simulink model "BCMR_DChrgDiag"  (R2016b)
settings: Solver=FixedStepDiscrete  StartTime=0.0  StopTime=10  FixedStep=0.01  RelTol=1e-3  EnableMultiTasking=on
undefined symbols (not defined in the file or in its folder): BCMR_bDChrgStopCActiveSw_C, BCMR_cntDChrgTCnntMax_C, BCMR_cntIsoFltTrigger_CW, BCMR_EVCCDiagccSw_C, BCMR_EVCCDiagSw_C, BCMR_G1E0PlatformSwDiag_C, BCMR_H1U0PlatformSwDiag_C, BCMR_iDcChrgDiffOvrCurr_C, BCMR_iDcChrgLowTempDiffOvrCurrMody_C, BCMR_iDcChrgLowTempOvrCurrCutOff_C, BCMR_iDcChrgLowTempOvrCurrHeal_C, BCMR_iDcChrgOvrCurr_C, BCMR_iDcChrgOvrVolt_C, BCMR_iDChrgCurrDiagLmt_C, BCMR_iDChrgCutOffVoltOvrCurrDet_C, BCMR_iDChrgCutOffVoltOvrCurrHeal_C, BCMR_kWaveFltFactor_C, BCMR_stCCSTimeout_C, BCMR_stCHMTimeout_C, BCMR_stCMLTimeout_C, BCMR_stCRMAATimeout_C, BCMR_stCROAATimeout_C, BCMR_stCROTimeout_C, BCMR_stCSDTimeout1_C, BCMR_stCSDTimeout2_C, BCMR_stCSTTimeout_C, BCMR_stCurrDwnTimeout_C, BCMR_stHvOnTimeout_C, BCMR_stNoTimeout_C, BCMR_stParaMish_C, BCMR_tBattLowTempDiagTempThrd_C, BCMR_tDcChrgIntfTempDiffLmt_C, BCMR_tDcChrgIntfTempLmt_C, BCMR_tiDChrgDetDiagDebs_C, BCMR_tiDChrgDetSec_C, BCMR_tiDChrgDiagBase_C, BCMR_tiDChrgHealDiagDebs_C, BCMR_tiDChrgIntfTempDwnLmt_C, BCMR_tiDChrgLowTOvrCurrDet_C, BCMR_tiDChrgLowTOvrCurrHeal_C, BCMR_tiDChrgMishCurrDetDiagDebs_C, BCMR_tiDChrgOvrCellVolt_C, BCMR_tiDChrgOvrSafeCellVoltDet_C, BCMR_tiDChrgVoltFltDetDebs_C, BCMR_tiDChrgVoltFltHealDebs_C, BCMR_uCC2ChkDiffDet_C, BCMR_uCC2ChkDiffHeal_C, BCMR_uCC2VoltHighDet_C, BCMR_uCC2VoltHighHeal_C, BCMR_uCC2VoltLowDet_C, BCMR_uCC2VoltLowHeal_C, BCMR_uDChrgHighTempDet_C, BCMR_uDChrgHighTempHeal_C, BCMR_uDChrgLowTempDet_C, BCMR_uDChrgLowTempHeal_C, BCMR_uDChrgOvrCellVoltDet_C, BCMR_uDChrgOvrCellVoltHeal_C, BCMR_uDChrgOvrSafeCellVoltDet_C, BCMR_uDChrgOvrSafeCellVoltHeal_C, bin2dec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
libraries: simulink x291
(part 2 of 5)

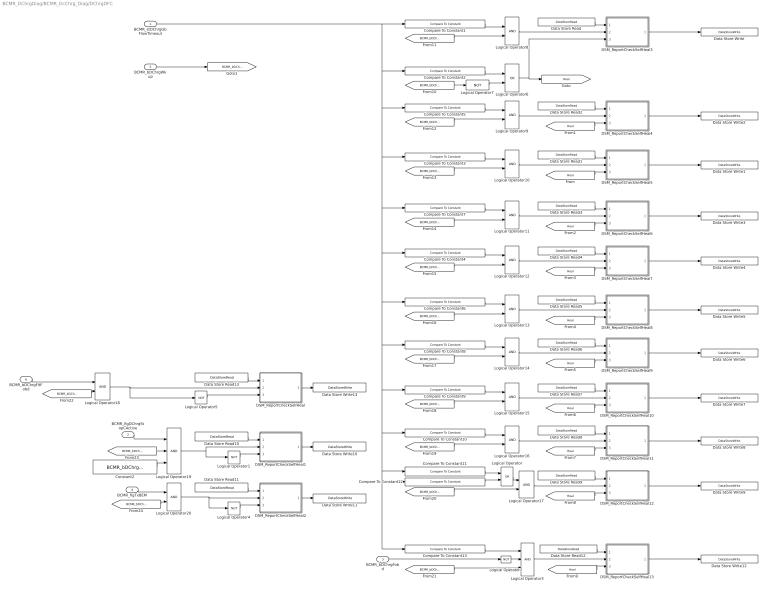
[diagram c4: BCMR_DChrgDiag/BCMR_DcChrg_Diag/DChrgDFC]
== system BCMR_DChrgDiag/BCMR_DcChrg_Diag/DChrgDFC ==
  BCMR_stDChrgGbFlowTimeout : Inport
  BCMR_flgDChrgStopCActive : Inport  Port=2
  BCMR_bDChrgFobd : Inport  Port=3
  BCMR_flgTxBEM : Inport  Port=4
  BCMR_bDChrgWkup : Inport  Port=5
  BCMR_bDChrgFltFobd : Inport  Port=6
  Compare To Constant1 : simulink/Logic and Bit Operations/Compare To Constant  relop===  const=BCMR_stCHMTimeout_C  OutDataTypeStr=boolean
  Compare To Constant10 : simulink/Logic and Bit Operations/Compare To Constant  relop===  const=BCMR_stCurrDwnTimeout_C  OutDataTypeStr=boolean
  Compare To Constant11 : simulink/Logic and Bit Operations/Compare To Constant  relop===  const=BCMR_stCSDTimeout1_C  OutDataTypeStr=boolean
  Compare To Constant12 : simulink/Logic and Bit Operations/Compare To Constant  relop===  const=BCMR_stCSDTimeout2_C  OutDataTypeStr=boolean
  Compare To Constant13 : simulink/Logic and Bit Operations/Compare To Constant  relop===  const=BCMR_stParaMish_C  OutDataTypeStr=boolean
  Compare To Constant2 : simulink/Logic and Bit Operations/Compare To Constant  relop===  const=BCMR_stNoTimeout_C  OutDataTypeStr=boolean
  Compare To Constant3 : simulink/Logic and Bit Operations/Compare To Constant  relop===  const=BCMR_stCRMAATimeout_C  OutDataTypeStr=boolean
  Compare To Constant4 : simulink/Logic and Bit Operations/Compare To Constant  relop===  const=BCMR_stCROTimeout_C  OutDataTypeStr=boolean
  Compare To Constant5 : simulink/Logic and Bit Operations/Compare To Constant  relop===  const=BCMR_stCMLTimeout_C  OutDataTypeStr=boolean
  Compare To Constant6 : simulink/Logic and Bit Operations/Compare To Constant  relop===  const=BCMR_stCROAATimeout_C  OutDataTypeStr=boolean
  Compare To Constant7 : simulink/Logic and Bit Operations/Compare To Constant  relop===  const=BCMR_stHvOnTimeout_C  OutDataTypeStr=boolean
  Compare To Constant8 : simulink/Logic and Bit Operations/Compare To Constant  relop===  const=BCMR_stCCSTimeout_C  OutDataTypeStr=boolean
  Compare To Constant9 : simulink/Logic and Bit Operations/Compare To Constant  relop===  const=BCMR_stCSTTimeout_C  OutDataTypeStr=boolean
  Constant2 : Constant  Value=BCMR_bDChrgStopCActiveSw_C
  DSM_ReportCheckSelfHeal : Subsystem  TreatAsAtomicUnit=on  RTWFcnName=DSM_ReportCheck  RTWFileName=SrvLib
  DSM_ReportCheckSelfHeal1 : Subsystem  TreatAsAtomicUnit=on  RTWFcnName=DSM_ReportCheck  RTWFileName=SrvLib
  DSM_ReportCheckSelfHeal10 : Subsystem  TreatAsAtomicUnit=on  RTWFcnName=DSM_ReportCheck  RTWFileName=SrvLib
  DSM_ReportCheckSelfHeal11 : Subsystem  TreatAsAtomicUnit=on  RTWFcnName=DSM_ReportCheck  RTWFileName=SrvLib
  DSM_ReportCheckSelfHeal12 : Subsystem  TreatAsAtomicUnit=on  RTWFcnName=DSM_ReportCheck  RTWFileName=SrvLib
  DSM_ReportCheckSelfHeal13 : Subsystem  TreatAsAtomicUnit=on  RTWFcnName=DSM_ReportCheck  RTWFileName=SrvLib
  DSM_ReportCheckSelfHeal2 : Subsystem  TreatAsAtomicUnit=on  RTWFcnName=DSM_ReportCheck  RTWFileName=SrvLib
  DSM_ReportCheckSelfHeal3 : Subsystem  TreatAsAtomicUnit=on  RTWFcnName=DSM_ReportCheck  RTWFileName=SrvLib
  DSM_ReportCheckSelfHeal4 : Subsystem  TreatAsAtomicUnit=on  RTWFcnName=DSM_ReportCheck  RTWFileName=SrvLib
  DSM_ReportCheckSelfHeal5 : Subsystem  TreatAsAtomicUnit=on  RTWFcnName=DSM_ReportCheck  RTWFileName=SrvLib
  DSM_ReportCheckSelfHeal6 : Subsystem  TreatAsAtomicUnit=on  RTWFcnName=DSM_ReportCheck  RTWFileName=SrvLib
  DSM_ReportCheckSelfHeal7 : Subsystem  TreatAsAtomicUnit=on  RTWFcnName=DSM_ReportCheck  RTWFileName=SrvLib
  DSM_ReportCheckSelfHeal8 : Subsystem  TreatAsAtomicUnit=on  RTWFcnName=DSM_ReportCheck  RTWFileName=SrvLib
  DSM_ReportCheckSelfHeal9 : Subsystem  TreatAsAtomicUnit=on  RTWFcnName=DSM_ReportCheck  RTWFileName=SrvLib
  Data Store Read : DataStoreRead  DataStoreName=DFC_DChrgCHMTmt
  Data Store Read1 : DataStoreRead  DataStoreName=DFC_DChrgCRMTmt
  Data Store Read10 : DataStoreRead  DataStoreName=DFC_DChrgStakeErr
  Data Store Read11 : DataStoreRead  DataStoreName=DFC_DChrgMsgTmt
  Data Store Read12 : DataStoreRead  DataStoreName=DFC_DChrgParaChk
  Data Store Read13 : DataStoreRead  DataStoreName=DFC_DChrgFobd
  Data Store Read2 : DataStoreRead  DataStoreName=DFC_DChrgCMLTmt
  Data Store Read3 : DataStoreRead  DataStoreName=DFC_DChrgHvOnFail
  Data Store Read4 : DataStoreRead  DataStoreName=DFC_DChrgCROTmt
  Data Store Read5 : DataStoreRead  DataStoreName=DFC_DChrgStkVoltErr
  Data Store Read6 : DataStoreRead  DataStoreName=DFC_DChrgCCSTmt
  Data Store Read7 : DataStoreRead  DataStoreName=DFC_DChrgCSTTmt
  Data Store Read8 : DataStoreRead  DataStoreName=DFC_DChrgStkCurrErr
  Data Store Read9 : DataStoreRead  DataStoreName=DFC_DChrgCSDTmt
  Data Store Write : DataStoreWrite  DataStoreName=DFC_DChrgCHMTmt
  Data Store Write1 : DataStoreWrite  DataStoreName=DFC_DChrgCRMTmt
  Data Store Write10 : DataStoreWrite  DataStoreName=DFC_DChrgStakeErr
  Data Store Write11 : DataStoreWrite  DataStoreName=DFC_DChrgMsgTmt
  Data Store Write12 : DataStoreWrite  DataStoreName=DFC_DChrgParaChk
  Data Store Write13 : DataStoreWrite  DataStoreName=DFC_DChrgFobd
  Data Store Write2 : DataStoreWrite  DataStoreName=DFC_DChrgCMLTmt
  Data Store Write3 : DataStoreWrite  DataStoreName=DFC_DChrgHvOnFail
  Data Store Write4 : DataStoreWrite  DataStoreName=DFC_DChrgCROTmt
  Data Store Write5 : DataStoreWrite  DataStoreName=DFC_DChrgStkVoltErr
  Data Store Write6 : DataStoreWrite  DataStoreName=DFC_DChrgCCSTmt
  Data Store Write7 : DataStoreWrite  DataStoreName=DFC_DChrgCSTTmt
  Data Store Write8 : DataStoreWrite  DataStoreName=DFC_DChrgStkCurrErr
  Data Store Write9 : DataStoreWrite  DataStoreName=DFC_DChrgCSDTmt
  Logical Operator : Logic  Operator=OR  AllPortsSameDT=off  OutDataTypeStr=boolean
  Logical Operator{1..2,4..5,7} (5 alike) : Logic  Operator=NOT  AllPortsSameDT=off  OutDataTypeStr=boolean
  Logical Operator{8..18,20} (12 alike) : Logic  AllPortsSameDT=off  OutDataTypeStr=boolean
  Logical Operator19 : Logic  Inputs=3  AllPortsSameDT=off  OutDataTypeStr=boolean
  Logical Operator3 : Logic  Inputs=3  AllPortsSameDT=off  OutDataTypeStr=boolean
  Logical Operator6 : Logic  Operator=OR  AllPortsSameDT=off  OutDataTypeStr=boolean
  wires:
  DSM_ReportCheckSelfHeal3/1(Dfc_id) -> Data Store Write/1
  Data Store Read/1 -> DSM_ReportCheckSelfHeal3/1(Dfc_id_nv)
  DSM_ReportCheckSelfHeal5/1(Dfc_id) -> Data Store Write1/1
  Data Store Read1/1 -> DSM_ReportCheckSelfHeal5/1(Dfc_id_nv)
  DSM_ReportCheckSelfHeal4/1(Dfc_id) -> Data Store Write2/1
  DSM_ReportCheckSelfHeal6/1(Dfc_id) -> Data Store Write3/1
  Data Store Read2/1 -> DSM_ReportCheckSelfHeal4/1(Dfc_id_nv)
  Data Store Read3/1 -> DSM_ReportCheckSelfHeal6/1(Dfc_id_nv)
  [Heal] -> DSM_ReportCheckSelfHeal5/3(Heal)
  [Heal] -> DSM_ReportCheckSelfHeal4/3(Heal)
  [Heal] -> DSM_ReportCheckSelfHeal6/3(Heal)
  DSM_ReportCheckSelfHeal7/1(Dfc_id) -> Data Store Write4/1
  Data Store Read4/1 -> DSM_ReportCheckSelfHeal7/1(Dfc_id_nv)
  [Heal] -> DSM_ReportCheckSelfHeal7/3(Heal)
  DSM_ReportCheckSelfHeal8/1(Dfc_id) -> Data Store Write5/1
  Data Store Read5/1 -> DSM_ReportCheckSelfHeal8/1(Dfc_id_nv)
  [Heal] -> DSM_ReportCheckSelfHeal8/3(Heal)
  DSM_ReportCheckSelfHeal9/1(Dfc_id) -> Data Store Write6/1
  Data Store Read6/1 -> DSM_ReportCheckSelfHeal9/1(Dfc_id_nv)
  [Heal] -> DSM_ReportCheckSelfHeal9/3(Heal)
  BCMR_stDChrgGbFlowTimeout/1 -> Compare To Constant8/1, Compare To Constant13/1, Compare To Constant12/1, Compare To Constant11/1, Compare To Constant10/1, Compare To Constant9/1, Compare To Constant6/1, Compare To Constant4/1, Compare To Constant7/1, Compare To Constant3/1, Compare To Constant5/1, Compare To Constant2/1, Compare To Constant1/1
  DSM_ReportCheckSelfHeal10/1(Dfc_id) -> Data Store Write7/1
  Data Store Read7/1 -> DSM_ReportCheckSelfHeal10/1(Dfc_id_nv)
  [Heal] -> DSM_ReportCheckSelfHeal10/3(Heal)
  DSM_ReportCheckSelfHeal11/1(Dfc_id) -> Data Store Write8/1
  Data Store Read8/1 -> DSM_ReportCheckSelfHeal11/1(Dfc_id_nv)
  [Heal] -> DSM_ReportCheckSelfHeal11/3(Heal)
  DSM_ReportCheckSelfHeal12/1(Dfc_id) -> Data Store Write9/1
  Data Store Read9/1 -> DSM_ReportCheckSelfHeal12/1(Dfc_id_nv)
  [Heal] -> DSM_ReportCheckSelfHeal12/3(Heal)
  Compare To Constant11/1 -> Logical Operator/1
  Compare To Constant12/1 -> Logical Operator/2
  Logical Operator1/1 -> DSM_ReportCheckSelfHeal1/3(Heal)
  DSM_ReportCheckSelfHeal1/1(Dfc_id) -> Data Store Write10/1
  Data Store Read10/1 -> DSM_ReportCheckSelfHeal1/1(Dfc_id_nv)
  DSM_ReportCheckSelfHeal13/1(Dfc_id) -> Data Store Write12/1
  Data Store Read12/1 -> DSM_ReportCheckSelfHeal13/1(Dfc_id_nv)
  [Heal] -> DSM_ReportCheckSelfHeal13/3(Heal)
  Logical Operator3/1 -> DSM_ReportCheckSelfHeal13/2(Err)
  Compare To Constant13/1 -> Logical Operator3/1
  Logical Operator2/1 -> Logical Operator3/2
  Logical Operator4/1 -> DSM_ReportCheckSelfHeal2/3(Heal)
  DSM_ReportCheckSelfHeal2/1(Dfc_id) -> Data Store Write11/1
  Data Store Read11/1 -> DSM_ReportCheckSelfHeal2/1(Dfc_id_nv)
  Data Store Read13/1 -> DSM_ReportCheckSelfHeal/1(Dfc_id_nv)
  Logical Operator5/1 -> DSM_ReportCheckSelfHeal/3(Heal)
  DSM_ReportCheckSelfHeal/1(Dfc_id) -> Data Store Write13/1
  BCMR_bDChrgWkup/1 -> [BCMR_bDChrgWkup]
  Compare To Constant2/1 -> Logical Operator6/1
  [BCMR_bDChrgWkup] -> Logical Operator7/1
  Logical Operator6/1 -> DSM_ReportCheckSelfHeal3/3(Heal), [Heal]
  Logical Operator7/1 -> Logical Operator6/2
  Logical Operator8/1 -> DSM_ReportCheckSelfHeal3/2(Err)
  Compare To Constant1/1 -> Logical Operator8/1
  [BCMR_bDChrgWkup] -> Logical Operator8/2
  Logical Operator9/1 -> DSM_ReportCheckSelfHeal4/2(Err)
  Compare To Constant5/1 -> Logical Operator9/1
  [BCMR_bDChrgWkup] -> Logical Operator9/2
  Logical Operator10/1 -> DSM_ReportCheckSelfHeal5/2(Err)
  Compare To Constant3/1 -> Logical Operator10/1
  [BCMR_bDChrgWkup] -> Logical Operator10/2
  Logical Operator11/1 -> DSM_ReportCheckSelfHeal6/2(Err)
  Compare To Constant7/1 -> Logical Operator11/1
  [BCMR_bDChrgWkup] -> Logical Operator11/2
  Logical Operator12/1 -> DSM_ReportCheckSelfHeal7/2(Err)
  Compare To Constant4/1 -> Logical Operator12/1
  [BCMR_bDChrgWkup] -> Logical Operator12/2
  Logical Operator13/1 -> DSM_ReportCheckSelfHeal8/2(Err)
  Compare To Constant6/1 -> Logical Operator13/1
  [BCMR_bDChrgWkup] -> Logical Operator13/2
  Logical Operator14/1 -> DSM_ReportCheckSelfHeal9/2(Err)
  Compare To Constant8/1 -> Logical Operator14/1
  [BCMR_bDChrgWkup] -> Logical Operator14/2
  Logical Operator15/1 -> DSM_ReportCheckSelfHeal10/2(Err)
  Compare To Constant9/1 -> Logical Operator15/1
  [BCMR_bDChrgWkup] -> Logical Operator15/2
  Logical Operator16/1 -> DSM_ReportCheckSelfHeal11/2(Err)
  Compare To Constant10/1 -> Logical Operator16/1
  [BCMR_bDChrgWkup] -> Logical Operator16/2
  Logical Operator17/1 -> DSM_ReportCheckSelfHeal12/2(Err)
  Logical Operator/1 -> Logical Operator17/1
  [BCMR_bDChrgWkup] -> Logical Operator17/2
  [BCMR_bDChrgWkup] -> Logical Operator3/3
  [BCMR_bDChrgWkup] -> Logical Operator18/2
  Logical Operator18/1 -> DSM_ReportCheckSelfHeal/2(Err), Logical Operator5/1
  Logical Operator19/1 -> DSM_ReportCheckSelfHeal1/2(Err), Logical Operator1/1
  BCMR_flgDChrgStopCActive/1 -> Logical Operator19/1
  [BCMR_bDChrgWkup] -> Logical Operator19/2
  Logical Operator20/1 -> DSM_ReportCheckSelfHeal2/2(Err), Logical Operator4/1
  BCMR_flgTxBEM/1 -> Logical Operator20/1
  [BCMR_bDChrgWkup] -> Logical Operator20/2
  BCMR_bDChrgFobd/1 -> Logical Operator2/1
  BCMR_bDChrgFltFobd/1 -> Logical Operator18/1
  Constant2/1 -> Logical Operator19/3

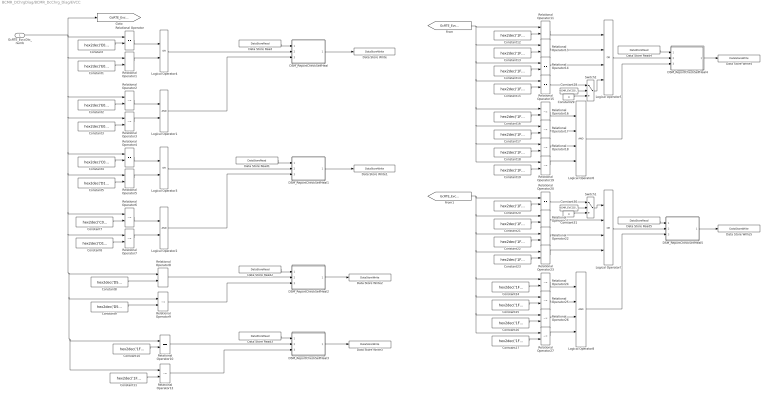
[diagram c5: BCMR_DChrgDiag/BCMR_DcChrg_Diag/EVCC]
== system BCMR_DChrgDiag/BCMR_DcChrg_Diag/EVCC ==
  GcRTE_EvccDtc_numb : Inport
  Constant : Constant  Value=hex2dec('E003')  OutDataTypeStr=uint16
  Constant1 : Constant  Value=hex2dec('E000')  OutDataTypeStr=uint16
  Constant10 : Constant  Value=hex2dec('1FF7')  OutDataTypeStr=uint16
  Constant11 : Constant  Value=hex2dec('1FF7')  OutDataTypeStr=uint16
  Constant12 : Constant  Value=hex2dec('1FF0')  OutDataTypeStr=uint16
  Constant13 : Constant  Value=hex2dec('1FF1')  OutDataTypeStr=uint16
  Constant14 : Constant  Value=hex2dec('1FF2')  OutDataTypeStr=uint16
  Constant{15,19..20,24} (4 alike) : Constant  Value=hex2dec('1FF4')  OutDataTypeStr=uint16
  Constant16 : Constant  Value=hex2dec('1FF0')  OutDataTypeStr=uint16
  Constant17 : Constant  Value=hex2dec('1FF1')  OutDataTypeStr=uint16
  Constant18 : Constant  Value=hex2dec('1FF2')  OutDataTypeStr=uint16
  Constant2 : Constant  Value=hex2dec('E003')  OutDataTypeStr=uint16
  Constant21 : Constant  Value=hex2dec('1FF5')  OutDataTypeStr=uint16
  Constant22 : Constant  Value=hex2dec('1FF6')  OutDataTypeStr=uint16
  Constant23 : Constant  Value=hex2dec('1FF8')  OutDataTypeStr=uint16
  Constant25 : Constant  Value=hex2dec('1FF5')  OutDataTypeStr=uint16
  Constant26 : Constant  Value=hex2dec('1FF6')  OutDataTypeStr=uint16
  Constant27 : Constant  Value=hex2dec('1FF8')  OutDataTypeStr=uint16
  Constant28 : Constant  Value=BCMR_EVCCDiagccSw_C
  Constant29 : Constant  Value=0
  Constant3 : Constant  Value=hex2dec('E000')  OutDataTypeStr=uint16
  Constant30 : Constant  Value=BCMR_EVCCDiagccSw_C
  Constant31 : Constant  Value=0
  Constant4 : Constant  Value=hex2dec('C078')  OutDataTypeStr=uint16
  Constant5 : Constant  Value=hex2dec('D111')  OutDataTypeStr=uint16
  Constant6 : Constant  Value=hex2dec('D111')  OutDataTypeStr=uint16
  Constant7 : Constant  Value=hex2dec('C078')  OutDataTypeStr=uint16
  Constant8 : Constant  Value=hex2dec('D563')  OutDataTypeStr=uint16
  Constant9 : Constant  Value=hex2dec('D563')  OutDataTypeStr=uint16
  DSM_ReportCheckSelfHeal : Subsystem  TreatAsAtomicUnit=on  RTWFcnName=DSM_ReportCheck  RTWFileName=SrvLib
  DSM_ReportCheckSelfHeal1 : Subsystem  TreatAsAtomicUnit=on  RTWFcnName=DSM_ReportCheck  RTWFileName=SrvLib
  DSM_ReportCheckSelfHeal2 : Subsystem  TreatAsAtomicUnit=on  RTWFcnName=DSM_ReportCheck  RTWFileName=SrvLib
  DSM_ReportCheckSelfHeal3 : Subsystem  TreatAsAtomicUnit=on  RTWFcnName=DSM_ReportCheck  RTWFileName=SrvLib
  DSM_ReportCheckSelfHeal4 : Subsystem  TreatAsAtomicUnit=on  RTWFcnName=DSM_ReportCheck  RTWFileName=SrvLib
  DSM_ReportCheckSelfHeal5 : Subsystem  TreatAsAtomicUnit=on  RTWFcnName=DSM_ReportCheck  RTWFileName=SrvLib
  Data Store Read : DataStoreRead  DataStoreName=DFC_EVCCDevFlt
  Data Store Read1 : DataStoreRead  DataStoreName=DFC_EVCCVehComFlt
  Data Store Read2 : DataStoreRead  DataStoreName=DFC_EVCCSplyPwrFlt
  Data Store Read3 : DataStoreRead  DataStoreName=DFC_EVCCPileComFlt
  Data Store Read4 : DataStoreRead  DataStoreName=DFC_EVCCPileHwFlt
  Data Store Read5 : DataStoreRead  DataStoreName=DFC_EVCCVehHwFlt
  Data Store Write : DataStoreWrite  DataStoreName=DFC_EVCCDevFlt
  Data Store Write1 : DataStoreWrite  DataStoreName=DFC_EVCCVehComFlt
  Data Store Write2 : DataStoreWrite  DataStoreName=DFC_EVCCSplyPwrFlt
  Data Store Write3 : DataStoreWrite  DataStoreName=DFC_EVCCPileComFlt
  Data Store Write4 : DataStoreWrite  DataStoreName=DFC_EVCCPileHwFlt
  Data Store Write5 : DataStoreWrite  DataStoreName=DFC_EVCCVehHwFlt
  Logical Operator1 : Logic  AllPortsSameDT=off  OutDataTypeStr=boolean
  Logical Operator2 : Logic  AllPortsSameDT=off  OutDataTypeStr=boolean
  Logical Operator3 : Logic  Operator=OR  AllPortsSameDT=off  OutDataTypeStr=boolean
  Logical Operator4 : Logic  Operator=OR  AllPortsSameDT=off  OutDataTypeStr=boolean
  Logical Operator5 : Logic  Operator=OR  Inputs=4  AllPortsSameDT=off  OutDataTypeStr=boolean
  Logical Operator6 : Logic  Inputs=4  AllPortsSameDT=off  OutDataTypeStr=boolean
  Logical Operator7 : Logic  Operator=OR  Inputs=4  AllPortsSameDT=off  OutDataTypeStr=boolean
  Logical Operator8 : Logic  Inputs=4  AllPortsSameDT=off  OutDataTypeStr=boolean
  Relational Operator{,1,4..5,8,10..11,13..15,20..23} (14 alike) : RelationalOperator  Operator===  OutDataTypeStr=boolean  RndMeth=Simplest
  Relational Operator{2..3,6..7,9,12,16..19,24..27} (14 alike) : RelationalOperator  Operator=~=  OutDataTypeStr=boolean  RndMeth=Simplest
  Switch1 : Switch  Criteria=u2 ~= 0
  Switch2 : Switch  Criteria=u2 ~= 0
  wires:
  DSM_ReportCheckSelfHeal/1(Dfc_id) -> Data Store Write/1
  Data Store Read/1 -> DSM_ReportCheckSelfHeal/1(Dfc_id_nv)
  Constant/1 -> Relational Operator/2
  Relational Operator/1 -> Logical Operator4/1
  Constant1/1 -> Relational Operator1/2
  Relational Operator1/1 -> Logical Operator4/2
  Logical Operator4/1 -> DSM_ReportCheckSelfHeal/2(Err)
  Relational Operator2/1 -> Logical Operator1/1
  Relational Operator3/1 -> Logical Operator1/2
  Constant2/1 -> Relational Operator2/2
  Constant3/1 -> Relational Operator3/2
  Logical Operator1/1 -> DSM_ReportCheckSelfHeal/3(Heal)
  Constant4/1 -> Relational Operator4/2
  Constant5/1 -> Relational Operator5/2
  Relational Operator5/1 -> Logical Operator3/2
  Logical Operator3/1 -> DSM_ReportCheckSelfHeal1/2(Err)
  Relational Operator6/1 -> Logical Operator2/1
  Relational Operator7/1 -> Logical Operator2/2
  Constant7/1 -> Relational Operator6/2
  Constant6/1 -> Relational Operator7/2
  Logical Operator2/1 -> DSM_ReportCheckSelfHeal1/3(Heal)
  Relational Operator4/1 -> Logical Operator3/1
  DSM_ReportCheckSelfHeal1/1(Dfc_id) -> Data Store Write1/1
  Data Store Read1/1 -> DSM_ReportCheckSelfHeal1/1(Dfc_id_nv)
  Data Store Read2/1 -> DSM_ReportCheckSelfHeal2/1(Dfc_id_nv)
  DSM_ReportCheckSelfHeal2/1(Dfc_id) -> Data Store Write2/1
  Constant8/1 -> Relational Operator8/2
  Relational Operator8/1 -> DSM_ReportCheckSelfHeal2/2(Err)
  Constant9/1 -> Relational Operator9/2
  Relational Operator9/1 -> DSM_ReportCheckSelfHeal2/3(Heal)
  Data Store Read3/1 -> DSM_ReportCheckSelfHeal3/1(Dfc_id_nv)
  DSM_ReportCheckSelfHeal3/1(Dfc_id) -> Data Store Write3/1
  Relational Operator10/1 -> DSM_ReportCheckSelfHeal3/2(Err)
  Relational Operator12/1 -> DSM_ReportCheckSelfHeal3/3(Heal)
  GcRTE_EvccDtc_numb/1 -> [GcRTE_EvccDtc_numb], Relational Operator3/1, Relational Operator12/1, Relational Operator10/1, Relational Operator9/1, Relational Operator8/1, Relational Operator7/1, Relational Operator6/1, Relational Operator5/1, Relational Operator4/1, Relational Operator2/1, Relational Operator1/1, Relational Operator/1
  Constant10/1 -> Relational Operator10/2
  Constant11/1 -> Relational Operator12/2
  DSM_ReportCheckSelfHeal4/1(Dfc_id) -> Data Store Write4/1
  Data Store Read4/1 -> DSM_ReportCheckSelfHeal4/1(Dfc_id_nv)
  Logical Operator6/1 -> DSM_ReportCheckSelfHeal4/3(Heal)
  Constant12/1 -> Relational Operator11/2
  Relational Operator11/1 -> Logical Operator5/1
  Constant13/1 -> Relational Operator13/2
  Relational Operator13/1 -> Logical Operator5/2
  [GcRTE_EvccDtc_numb] -> Relational Operator19/1, Relational Operator18/1, Relational Operator17/1, Relational Operator16/1, Relational Operator15/1, Relational Operator14/1, Relational Operator13/1, Relational Operator11/1
  Logical Operator5/1 -> DSM_ReportCheckSelfHeal4/2(Err)
  Relational Operator14/1 -> Logical Operator5/3
  Constant14/1 -> Relational Operator14/2
  Constant15/1 -> Relational Operator15/2
  Relational Operator19/1 -> Logical Operator6/4
  Relational Operator18/1 -> Logical Operator6/3
  Relational Operator17/1 -> Logical Operator6/2
  Relational Operator16/1 -> Logical Operator6/1
  Constant16/1 -> Relational Operator16/2
  Constant17/1 -> Relational Operator17/2
  Constant18/1 -> Relational Operator18/2
  Constant19/1 -> Relational Operator19/2
  DSM_ReportCheckSelfHeal5/1(Dfc_id) -> Data Store Write5/1
  Data Store Read5/1 -> DSM_ReportCheckSelfHeal5/1(Dfc_id_nv)
  Logical Operator8/1 -> DSM_ReportCheckSelfHeal5/3(Heal)
  Constant20/1 -> Relational Operator20/2
  Constant21/1 -> Relational Operator21/2
  Relational Operator21/1 -> Logical Operator7/2
  [GcRTE_EvccDtc_numb] -> Relational Operator20/1, Relational Operator21/1, Relational Operator22/1, Relational Operator23/1, Relational Operator24/1, Relational Operator25/1, Relational Operator26/1, Relational Operator27/1
  Logical Operator7/1 -> DSM_ReportCheckSelfHeal5/2(Err)
  Relational Operator22/1 -> Logical Operator7/3
  Constant22/1 -> Relational Operator22/2
  Relational Operator23/1 -> Logical Operator7/4
  Constant23/1 -> Relational Operator23/2
  Relational Operator27/1 -> Logical Operator8/4
  Relational Operator26/1 -> Logical Operator8/3
  Relational Operator25/1 -> Logical Operator8/2
  Relational Operator24/1 -> Logical Operator8/1
  Constant24/1 -> Relational Operator24/2
  Constant25/1 -> Relational Operator25/2
  Constant26/1 -> Relational Operator26/2
  Constant27/1 -> Relational Operator27/2
  Relational Operator15/1 -> Switch2/1
  Constant28/1 -> Switch2/2
  Constant29/1 -> Switch2/3
  Switch2/1 -> Logical Operator5/4
  Constant30/1 -> Switch1/2
  Constant31/1 -> Switch1/3
  Switch1/1 -> Logical Operator7/1
  Relational Operator20/1 -> Switch1/1

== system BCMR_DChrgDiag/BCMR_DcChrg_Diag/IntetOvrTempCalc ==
  BSPR_tDcChNeg : Inport
  BSPR_tDcChPos : Inport  Port=2
  COMR_tEnvT : Inport  Port=3
  BCMR_bDChrgWkup : Inport  Port=4
  DChrgInletDiag : Subsystem
  Subsystem : Subsystem
  BCMR_stDcOutpCnntOvrTempErr : Outport  OutputWhenDisabled=reset  InitialOutput=[0]
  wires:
  BSPR_tDcChNeg/1 -> DChrgInletDiag/1(BSPR_tDcChNeg)
  BSPR_tDcChPos/1 -> DChrgInletDiag/2(BSPR_tDcChPos)
  COMR_tEnvT/1 -> DChrgInletDiag/3(COMR_tEnvT)
  DChrgInletDiag/1(BCMR_stDcOutpCnntOvrTempDet) -> Subsystem/1(BCMR_stDcOutpCnntOvrTempDet)
  DChrgInletDiag/2(BCMR_stDcOutpCnntOvrTempHeal) -> Subsystem/2(BCMR_stDcOutpCnntOvrTempHeal)
  Subsystem/1(BCMR_stDcOutpCnntOvrTempErr) -> BCMR_stDcOutpCnntOvrTempErr/1
  BCMR_bDChrgWkup/1 -> DChrgInletDiag/Enable

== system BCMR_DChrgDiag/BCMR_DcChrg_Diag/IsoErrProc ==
  HVSR_flgIsoFaultLvl2 : Inport
  Constant : Constant  OutDataTypeStr=uint8
  Constant1 : Constant  Value=0  OutDataTypeStr=uint8
  Constant2 : Constant  Value=BCMR_cntIsoFltTrigger_CW  OutDataTypeStr=uint8
  Constant3 : Constant  OutDataTypeStr=uint8
  Switch : Switch  Criteria=u2 > Threshold
  Switch1 : Switch  Criteria=u2 > Threshold  Threshold=77
  BCMR_stDcBattInsulationErr : Outport
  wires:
  Constant1/1 -> Switch/3
  HVSR_flgIsoFaultLvl2/1 -> Switch/2
  Constant/1 -> Switch/1
  Switch/1 -> Switch1/1
  Constant2/1 -> Switch1/2
  Constant3/1 -> Switch1/3
  Switch1/1 -> BCMR_stDcBattInsulationErr/1  "BCMR_stDcBattInsulationErr"

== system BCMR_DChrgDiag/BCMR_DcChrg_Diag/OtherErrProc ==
  COMR_stVcuFalutLvl : Inport
  DSMR_stFaultRank : Inport  Port=2
  HVSR_flgHvilFault : Inport  Port=3
  BCMR_bDcComErrDet : Inport  Port=4
  COMR_stPwrUpDwnVcuReq : Inport  Port=5
  BCMR_stDChrgMode : Inport  Port=6
  Compare To Constant : simulink/Logic and Bit Operations/Compare To Constant  relop=>=  const=3  OutDataTypeStr=uint8
  Compare To Constant1 : simulink/Logic and Bit Operations/Compare To Constant  relop===  const=3  OutDataTypeStr=boolean
  Compare To Constant13 : simulink/Logic and Bit Operations/Compare To Constant  relop===  const=2  OutDataTypeStr=boolean
  Compare To Constant2 : simulink/Logic and Bit Operations/Compare To Constant  relop===  const=4  OutDataTypeStr=boolean
  Compare To Constant6 : simulink/Logic and Bit Operations/Compare To Constant  relop=>=  const=3  OutDataTypeStr=boolean
  Constant5 : Constant  Value=BCMR_tiDChrgDetDiagDebs_C
  Constant7 : Constant  Value=BCMR_tiDChrgDiagBase_C
  Data Type Conversion : DataTypeConversion  OutDataTypeStr=uint8
  Logical Operator2 : Logic  Operator=OR  Inputs=5  AllPortsSameDT=off  OutDataTypeStr=boolean
  Logical Operator3 : Logic  AllPortsSameDT=off  OutDataTypeStr=boolean
  Logical Operator4 : Logic  Operator=OR  AllPortsSameDT=off  OutDataTypeStr=boolean
  TONV_VariableTimeDebounce : Subsystem  TreatAsAtomicUnit=on  RTWFcnName=TONV_VariableTimeDebounce  RTWFileName=SrvLib
  BCMR_stOtherErr : Outport
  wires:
  COMR_stVcuFalutLvl/1 -> Compare To Constant/1
  Data Type Conversion/1 -> BCMR_stOtherErr/1  "BCMR_stOtherErr"
  Constant7/1 -> TONV_VariableTimeDebounce/3(dT)
  Constant5/1 -> TONV_VariableTimeDebounce/2(T)
  Compare To Constant/1 -> TONV_VariableTimeDebounce/1(u)
  Logical Operator2/1 -> Data Type Conversion/1
  TONV_VariableTimeDebounce/1(y) -> Logical Operator2/1
  DSMR_stFaultRank/1 -> Compare To Constant6/1
  Compare To Constant6/1 -> Logical Operator2/3
  HVSR_flgHvilFault/1 -> Logical Operator2/2
  BCMR_bDcComErrDet/1 -> Logical Operator2/4
  COMR_stPwrUpDwnVcuReq/1 -> Compare To Constant13/1
  BCMR_stDChrgMode/1 -> Compare To Constant2/1, Compare To Constant1/1
  Logical Operator3/1 -> Logical Operator2/5
  Compare To Constant13/1 -> Logical Operator3/1
  Compare To Constant1/1 -> Logical Operator4/1
  Logical Operator4/1 -> Logical Operator3/2
  Compare To Constant2/1 -> Logical Operator4/2

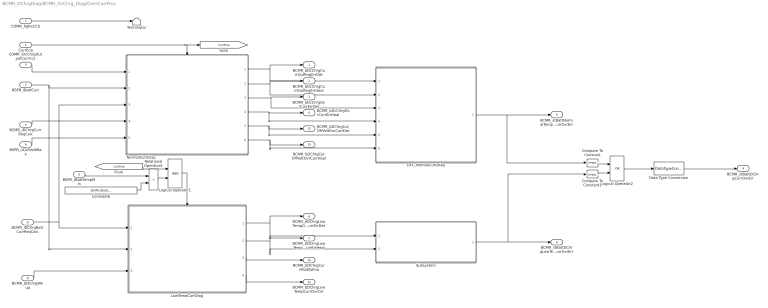
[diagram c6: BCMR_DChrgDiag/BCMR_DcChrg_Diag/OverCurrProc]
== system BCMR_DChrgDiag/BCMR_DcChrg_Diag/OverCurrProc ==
  CurrEna : Inport
  BSPR_iBattCurr : Inport  Port=2
  COMR_iDcChrgOutputCurrCcs : Inport  Port=3
  BCMR_iDChrgCurrReqCalc : Inport  Port=4
  BSPR_tBattTempMin : Inport  Port=5
  BCMR_iDChrgBattCurrReqCalc : Inport  Port=6
  COMR_flgRxCCS : Inport  Port=7
  BCMR_bDChrgWkup : Inport  Port=8
  BSPR_uCellVoltMax : Inport  Port=9
  Compare To Constant : simulink/Logic and Bit Operations/Compare To Constant  relop=>  const=0  OutDataTypeStr=boolean
  Compare To Constant1 : simulink/Logic and Bit Operations/Compare To Constant  relop=>  const=0  OutDataTypeStr=boolean
  Constant6 : Constant  Value=BCMR_tBattLowTempDiagTempThrd_C  OutDataTypeStr=single
  DFC_NormalCurrDiag : Subsystem
  Data Type Conversion : DataTypeConversion  OutDataTypeStr=uint8
  Logical Operator1 : Logic  AllPortsSameDT=off  OutDataTypeStr=boolean
  Logical Operator2 : Logic  Operator=OR  AllPortsSameDT=off  OutDataTypeStr=boolean
  LowTempCurrDiag : Subsystem
  NormalCurrDiag : Subsystem
  Relational Operator4 : RelationalOperator  Operator=<  OutDataTypeStr=boolean  RndMeth=Simplest
  Subsystem : Subsystem
  Terminator : Terminator
  BCMR_bDcChrgCurrOutRngErrDet : Outport
  BCMR_bDcChrgCurrOutRngErrHeal : Outport  Port=2
  BCMR_bDcChrgOvrCurrErrDet : Outport  Port=3
  BCMR_bDcChrgOvrCurrErrHeal : Outport  Port=4
  BCMR_stBattNormalTempDChrgCurrOvrErr : Outport  Port=5  OutputWhenDisabled=reset  InitialOutput=[0]
  BCMR_bDChrgLowTempOvrCurrErrDet : Outport  Port=6  InitialOutput=[0]
  BCMR_bDChrgLowTempOvrCurrErrHeal : Outport  Port=7  InitialOutput=[0]
  BCMR_stBattDChrgLowTempCurrOvrErr : Outport  Port=8  OutputWhenDisabled=reset  InitialOutput=[0]
  BCMR_stBattDChrgCurrOvrErr : Outport  Port=9  OutputWhenDisabled=reset  InitialOutput=[0]
  BCMR_bDChrgCurrModifyEna : Outport  Port=10  InitialOutput=[0]
  BCMR_bDChrgLowTempCurrOvrCnt : Outport  Port=11  OutputWhenDisabled=reset  InitialOutput=[0]
  BCMR_bDChrgCutOffVoltOvrCurrDet : Outport  Port=12
  BCMR_bDChrgCutOffVoltOvrCurrHeal : Outport  Port=13
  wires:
  BSPR_iBattCurr/1 -> NormalCurrDiag/2(BSPR_iBattCurr), LowTempCurrDiag/2(BSPR_iBattCurr)
  BCMR_iDChrgCurrReqCalc/1 -> NormalCurrDiag/4(BCMR_iDChrgCurrReqCalc)
  NormalCurrDiag/1(BCMR_bDcChrgCurrOutRngErrDet) -> DFC_NormalCurrDiag/1(BCMR_bDcChrgCurrOutRngErrDet), BCMR_bDcChrgCurrOutRngErrDet/1
  NormalCurrDiag/2(BCMR_bDcChrgCurrOutRngErrHeal) -> DFC_NormalCurrDiag/2(BCMR_bDcChrgCurrOutRngErrHeal), BCMR_bDcChrgCurrOutRngErrHeal/1
  NormalCurrDiag/3(BCMR_bDcChrgOvrCurrErrDet) -> DFC_NormalCurrDiag/3(BCMR_bDcChrgOvrCurrErrDet), BCMR_bDcChrgOvrCurrErrDet/1
  NormalCurrDiag/4(BCMR_bDcChrgOvrCurrErrHeal) -> DFC_NormalCurrDiag/4(BCMR_bDcChrgOvrCurrErrHeal), BCMR_bDcChrgOvrCurrErrHeal/1
  BCMR_iDChrgBattCurrReqCalc/1 -> LowTempCurrDiag/1(BCMR_iDChrgBattCurrReqCalc), NormalCurrDiag/3(BCMR_iDChrgBattCurrReqCalc)
  LowTempCurrDiag/1(BCMR_bDChrgLowTempOvrCurrErrDet) -> Subsystem/1(BCMR_bDChrgLowTempOvrCurrErrDet), BCMR_bDChrgLowTempOvrCurrErrDet/1
  LowTempCurrDiag/2(BCMR_bDChrgLowTempOvrCurrErrHeal) -> Subsystem/2(BCMR_bDChrgLowTempOvrCurrErrHeal), BCMR_bDChrgLowTempOvrCurrErrHeal/1
  Compare To Constant/1 -> Logical Operator2/1
  Compare To Constant1/1 -> Logical Operator2/2
  Logical Operator2/1 -> Data Type Conversion/1
  Data Type Conversion/1 -> BCMR_stBattDChrgCurrOvrErr/1
  LowTempCurrDiag/3(BCMR_bDChrgLowTempCurrModifyEna) -> BCMR_bDChrgCurrModifyEna/1
  BCMR_bDChrgWkup/1 -> LowTempCurrDiag/3(BCMR_bDChrgWkup)
  LowTempCurrDiag/4(BCMR_bDChrgCurrOvrCnt) -> BCMR_bDChrgLowTempCurrOvrCnt/1
  BSPR_uCellVoltMax/1 -> NormalCurrDiag/5(BSPR_uCellVoltMax)
  NormalCurrDiag/5(BCMR_bDChrgCutOffVoltOvrCurrDet) -> DFC_NormalCurrDiag/5(BCMR_bDChrgCutOffVoltOvrCurrDet), BCMR_bDChrgCutOffVoltOvrCurrDet/1
  NormalCurrDiag/6(BCMR_bDChrgCutOffVoltOvrCurrHeal) -> DFC_NormalCurrDiag/6(BCMR_bDChrgCutOffVoltOvrCurrHeal), BCMR_bDChrgCutOffVoltOvrCurrHeal/1
  COMR_iDcChrgOutputCurrCcs/1 -> NormalCurrDiag/1(COMR_iDcChrgOutputCurrCcs)
  COMR_flgRxCCS/1 -> Terminator/1
  DFC_NormalCurrDiag/1(BCMR_stBattNormalTempDChrgCurrOvrErr) -> Compare To Constant/1, BCMR_stBattNormalTempDChrgCurrOvrErr/1
  CurrEna/1 -> [CurrEna], NormalCurrDiag/Enable
  Logical Operator1/1 -> LowTempCurrDiag/Enable
  Subsystem/1(BCMR_stBattDChrgLowTempCurrOvrErr) -> Compare To Constant1/1, BCMR_stBattDChrgLowTempCurrOvrErr/1
  [CurrEna] -> Logical Operator1/1
  Relational Operator4/1 -> Logical Operator1/2
  BSPR_tBattTempMin/1 -> Relational Operator4/1
  Constant6/1 -> Relational Operator4/2

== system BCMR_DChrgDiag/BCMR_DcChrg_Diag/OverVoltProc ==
  BSPR_uCellVoltMax : Inport
  BSPR_uDChrgVolt : Inport  Port=2
  BSPR_uPackVolt : Inport  Port=3
  BSPR_uBattVolt : Inport  Port=4
  COMR_flgRxCCS : Inport  Port=5
  CurrEna : Inport  Port=6
  DChrgVoltDiag : Subsystem
  DFC_DChrgVoltDiag : Subsystem
  Terminator : Terminator
  BCMR_bDcChrgVoltOutRngErrHeal : Outport
  BCMR_bDcChrgVoltOutRngErrDet : Outport  Port=2
  BCMR_stBattDChrgVoltOvrErr : Outport  Port=3  OutputWhenDisabled=reset  InitialOutput=[0]
  BCMR_bDChrgOvrSafeCellVoltDet : Outport  Port=4
  BCMR_bDChrgOvrSafeCellVoltHeal : Outport  Port=5
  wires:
  COMR_flgRxCCS/1 -> Terminator/1
  BSPR_uCellVoltMax/1 -> DChrgVoltDiag/1(BSPR_uCellVoltMax)
  BSPR_uPackVolt/1 -> DChrgVoltDiag/3(BSPR_uPackVolt)
  BSPR_uBattVolt/1 -> DChrgVoltDiag/4(BSPR_uBattVolt)
  BSPR_uDChrgVolt/1 -> DChrgVoltDiag/2(BSPR_uDChrgVolt)
  DChrgVoltDiag/4(BCMR_bDcChrgVoltOutRngErrHeal) -> DFC_DChrgVoltDiag/4(BCMR_bDcChrgVoltOutRngErrHeal), BCMR_bDcChrgVoltOutRngErrHeal/1
  DChrgVoltDiag/3(BCMR_bDcChrgVoltOutRngErrDet) -> DFC_DChrgVoltDiag/3(BCMR_bDcChrgVoltOutRngErrDet), BCMR_bDcChrgVoltOutRngErrDet/1
  DChrgVoltDiag/1(BCMR_bDChrgOvrSafeCellVoltDet) -> DFC_DChrgVoltDiag/1(BCMR_bDChrgOvrSafeCellVoltDet), BCMR_bDChrgOvrSafeCellVoltDet/1
  DChrgVoltDiag/2(BCMR_bDChrgOvrSafeCellVoltHeal) -> DFC_DChrgVoltDiag/2(BCMR_bDChrgOvrSafeCellVoltHeal), BCMR_bDChrgOvrSafeCellVoltHeal/1
  CurrEna/1 -> DChrgVoltDiag/Enable
  DFC_DChrgVoltDiag/1(BCMR_stBattDChrgVoltOvrErr) -> BCMR_stBattDChrgVoltOvrErr/1

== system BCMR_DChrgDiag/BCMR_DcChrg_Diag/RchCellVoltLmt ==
  BCMR_flgDChrgFulChk : Inport
  BCMR_stDChrgMode : Inport  Port=2
  Enable : EnablePort  StatesWhenEnabling=reset
  Compare To Constant1 : simulink/Logic and Bit Operations/Compare To Constant  relop===  const=6  OutDataTypeStr=boolean
  Compare To Constant2 : simulink/Logic and Bit Operations/Compare To Constant  relop===  const=0  OutDataTypeStr=boolean
  Constant1 : Constant  OutDataTypeStr=uint8
  Constant5 : Constant  Value=0  OutDataTypeStr=uint8
  Logical Operator : Logic  Operator=OR  AllPortsSameDT=off  OutDataTypeStr=boolean
  Subsystem3 : Subsystem
  Switch : Switch  Criteria=u2 > Threshold  OutDataTypeStr=uint8
  BCMR_stDcRchCellVoltLmt : Outport  OutDataTypeStr=uint8  OutputWhenDisabled=reset  InitialOutput=[0]
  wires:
  Constant1/1 -> Switch/1
  Constant5/1 -> Switch/3
  Switch/1 -> BCMR_stDcRchCellVoltLmt/1
  BCMR_stDChrgMode/1 -> Compare To Constant2/1, Compare To Constant1/1
  Compare To Constant2/1 -> Logical Operator/2
  Compare To Constant1/1 -> Logical Operator/1
  Logical Operator/1 -> Subsystem3/2(clear)
  BCMR_flgDChrgFulChk/1 -> Subsystem3/1(set)
  Subsystem3/1(Q) -> Switch/2

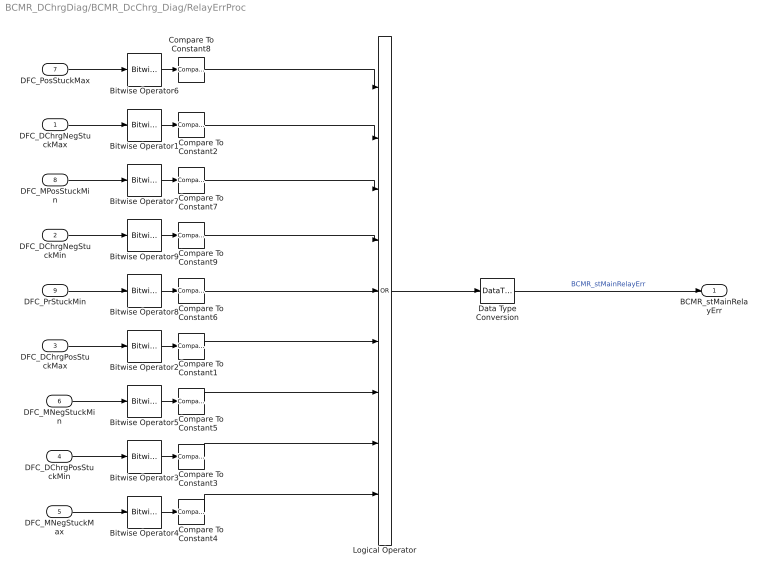
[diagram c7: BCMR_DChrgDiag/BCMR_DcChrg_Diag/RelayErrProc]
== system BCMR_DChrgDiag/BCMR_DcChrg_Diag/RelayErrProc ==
  DFC_DChrgNegStuckMax : Inport
  DFC_DChrgNegStuckMin : Inport  Port=2
  DFC_DChrgPosStuckMax : Inport  Port=3
  DFC_DChrgPosStuckMin : Inport  Port=4
  DFC_MNegStuckMax : Inport  Port=5
  DFC_MNegStuckMin : Inport  Port=6
  DFC_PosStuckMax : Inport  Port=7
  DFC_MPosStuckMin : Inport  Port=8
  DFC_PrStuckMin : Inport  Port=9
  Bitwise Operator{1..9} (9 alike) : simulink/Logic and Bit Operations/Bitwise Operator  logicop=AND  UseBitMask=on  BitMask=bin2dec('00011000')  BitMaskRealWorld=Stored Integer
  Compare To Constant{1..9} (9 alike) : simulink/Logic and Bit Operations/Compare To Constant  relop===  const=24  OutDataTypeStr=boolean
  Data Type Conversion : DataTypeConversion  OutDataTypeStr=uint8
  Logical Operator : Logic  Operator=OR  Inputs=9  AllPortsSameDT=off  OutDataTypeStr=boolean
  BCMR_stMainRelayErr : Outport
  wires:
  DFC_DChrgNegStuckMin/1 -> Bitwise Operator9/1
  DFC_DChrgPosStuckMax/1 -> Bitwise Operator2/1
  DFC_DChrgPosStuckMin/1 -> Bitwise Operator3/1
  DFC_MNegStuckMax/1 -> Bitwise Operator4/1
  DFC_MNegStuckMin/1 -> Bitwise Operator5/1
  DFC_PosStuckMax/1 -> Bitwise Operator6/1
  DFC_MPosStuckMin/1 -> Bitwise Operator7/1
  DFC_PrStuckMin/1 -> Bitwise Operator8/1
  Data Type Conversion/1 -> BCMR_stMainRelayErr/1  "BCMR_stMainRelayErr"
  Bitwise Operator2/1 -> Compare To Constant1/1
  Bitwise Operator3/1 -> Compare To Constant3/1
  Bitwise Operator4/1 -> Compare To Constant4/1
  Bitwise Operator5/1 -> Compare To Constant5/1
  Compare To Constant5/1 -> Logical Operator/7
  Bitwise Operator7/1 -> Compare To Constant7/1
  Bitwise Operator6/1 -> Compare To Constant8/1
  Logical Operator/1 -> Data Type Conversion/1
  Bitwise Operator1/1 -> Compare To Constant2/1
  DFC_DChrgNegStuckMax/1 -> Bitwise Operator1/1
  Bitwise Operator9/1 -> Compare To Constant9/1
  Bitwise Operator8/1 -> Compare To Constant6/1
  Compare To Constant8/1 -> Logical Operator/1
  Compare To Constant2/1 -> Logical Operator/2
  Compare To Constant7/1 -> Logical Operator/3
  Compare To Constant9/1 -> Logical Operator/4
  Compare To Constant6/1 -> Logical Operator/5
  Compare To Constant1/1 -> Logical Operator/6
  Compare To Constant3/1 -> Logical Operator/8
  Compare To Constant4/1 -> Logical Operator/9

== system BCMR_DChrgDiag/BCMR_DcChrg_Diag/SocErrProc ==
  DFC_SocRngHiMax : Inport
  DFC_SocRngHiMin : Inport  Port=2
  DFC_SocRngLoMax : Inport  Port=3
  DFC_SocRngLoMin : Inport  Port=4
  Bitwise Operator{1..4} (4 alike) : simulink/Logic and Bit Operations/Bitwise Operator  logicop=AND  UseBitMask=on  BitMask=bin2dec('00011000')  BitMaskRealWorld=Stored Integer
  Compare To Constant{,1..3} (4 alike) : simulink/Logic and Bit Operations/Compare To Constant  relop===  const=24  OutDataTypeStr=boolean
  Constant : Constant  OutDataTypeStr=uint8
  Constant9 : Constant  Value=2  OutDataTypeStr=uint8
  Delay : Delay  DelayLength=1  InitialCondition=0
  Logical Operator : Logic  Operator=OR  AllPortsSameDT=off  OutDataTypeStr=boolean
  Logical Operator1 : Logic  Operator=OR  AllPortsSameDT=off  OutDataTypeStr=boolean
  Switch4 : Switch  Criteria=u2 > Threshold
  Switch5 : Switch  Criteria=u2 > Threshold
  BCMR_stDcBattSocErr : Outport
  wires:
  DFC_SocRngHiMax/1 -> Bitwise Operator4/1
  DFC_SocRngHiMin/1 -> Bitwise Operator1/1
  DFC_SocRngLoMax/1 -> Bitwise Operator2/1
  DFC_SocRngLoMin/1 -> Bitwise Operator3/1
  Compare To Constant/1 -> Logical Operator/1
  Compare To Constant1/1 -> Logical Operator/2
  Compare To Constant2/1 -> Logical Operator1/1
  Compare To Constant3/1 -> Logical Operator1/2
  Constant/1 -> Switch4/1
  Logical Operator/1 -> Switch4/2
  Logical Operator1/1 -> Switch5/2
  Constant9/1 -> Switch5/1
  Switch5/1 -> Delay/1, Switch4/3
  Switch4/1 -> BCMR_stDcBattSocErr/1  "BCMR_stDcBattSocErr"
  Delay/1 -> Switch5/3
  Bitwise Operator4/1 -> Compare To Constant/1
  Bitwise Operator1/1 -> Compare To Constant1/1
  Bitwise Operator2/1 -> Compare To Constant2/1
  Bitwise Operator3/1 -> Compare To Constant3/1

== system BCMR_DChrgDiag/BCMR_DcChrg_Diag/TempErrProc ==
  BSPR_tBattTempMax : Inport
  BCMR_bDChrgWkup : Inport  Port=2
  DFC_BattTAlrmMax : Inport  Port=3
  DFC_BattTFaultMax : Inport  Port=4
  "DFC_BattTWarnMax " : Inport  Port=5
  DFC_BattTAlrmMin : Inport  Port=6
  DFC_BattTFaultMin : Inport  Port=7
  DFC_BattTWarnMin : Inport  Port=8
  BSPR_tBattTempMin : Inport  Port=9
  Subsystem : Subsystem
  Subsystem1 : Subsystem
  Terminator{1..4} (4 alike) : Terminator
  BCMR_bDChrgTempLowErrDet : Outport  OutputWhenDisabled=reset  InitialOutput=[0]
  BCMR_stDcBattTempOvrErr : Outport  Port=2
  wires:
  DFC_BattTAlrmMax/1 -> Terminator1/1
  DFC_BattTWarnMin/1 -> Terminator4/1
  DFC_BattTFaultMin/1 -> Terminator3/1
  DFC_BattTAlrmMin/1 -> Terminator2/1
  BSPR_tBattTempMin/1 -> Subsystem/1(BSPR_tBattTempMin)
  Subsystem/1(BCMR_bDChrgTempLowErrDet) -> BCMR_bDChrgTempLowErrDet/1, Subsystem1/3(BCMR_bDChrgTempLowErrDet)
  Subsystem/2(BCMR_bDChrgTempLowErrHeal) -> Subsystem1/4(BCMR_bDChrgTempLowErrHeal)
  DFC_BattTFaultMax/1 -> Subsystem1/1(DFC_BattTFaultMax)
  "DFC_BattTWarnMax "/1 -> Subsystem1/2("DFC_BattTWarnMax ")
  Subsystem1/1(BCMR_stDcBattTempOvrErr) -> BCMR_stDcBattTempOvrErr/1
  BCMR_bDChrgWkup/1 -> Subsystem/Enable
  BSPR_tBattTempMax/1 -> Subsystem/2(BSPR_tBattTempMax)
  Subsystem/3(BCMR_bDChrgTempHighErrDet) -> Subsystem1/5(BCMR_bDChrgTempHighErrDet)
  Subsystem/4(BCMR_bDChrgTempHighErrHeal) -> Subsystem1/6(BCMR_bDChrgTempHighErrHeal)

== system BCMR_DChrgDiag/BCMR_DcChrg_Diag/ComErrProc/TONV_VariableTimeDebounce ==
  note: Turn On Delay Time Deboune
  u : Inport
  T : Inport  Port=2
  dT : Inport  Port=3
  Add : Sum
  Constant1 : Constant  Value=0  OutDataTypeStr=single
  Constant2 : Constant  OutDataTypeStr=uint8
  Constant3 : Constant  Value=0  OutDataTypeStr=uint8
  Delay : Delay  DelayLength=1  InitialCondition=0
  MinMax : MinMax  Inputs=2
  Product : Product  OutMin=[0]  OutMax=[65535]  OutDataTypeStr=single
  Relational Operator : RelationalOperator  Operator=>  OutDataTypeStr=boolean  RndMeth=Simplest
  Switch : Switch  Criteria=u2 ~= 0
  Switch1 : Switch  Criteria=u2 ~= 0
  y : Outport
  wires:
  Switch1/1 -> Product/1
  Constant3/1 -> Switch1/3
  Constant2/1 -> Switch1/1
  u/1 -> Switch1/2, Switch/2
  dT/1 -> Switch/1
  Constant1/1 -> Switch/3
  Add/1 -> Product/2
  Product/1 -> Relational Operator/1, Delay/1
  Switch/1 -> Add/1
  Delay/1 -> MinMax/2
  Relational Operator/1 -> y/1
  T/1 -> MinMax/1, Relational Operator/2
  MinMax/1 -> Add/2

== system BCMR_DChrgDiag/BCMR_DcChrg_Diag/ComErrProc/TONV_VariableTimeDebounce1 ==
  note: Turn On Delay Time Deboune
  u : Inport
  T : Inport  Port=2
  dT : Inport  Port=3
  Add : Sum
  Constant1 : Constant  Value=0  OutDataTypeStr=single
  Constant2 : Constant  OutDataTypeStr=uint8
  Constant3 : Constant  Value=0  OutDataTypeStr=uint8
  Delay : Delay  DelayLength=1  InitialCondition=0
  MinMax : MinMax  Inputs=2
  Product : Product  OutMin=[0]  OutMax=[65535]  OutDataTypeStr=single
  Relational Operator : RelationalOperator  Operator=>  OutDataTypeStr=boolean  RndMeth=Simplest
  Switch : Switch  Criteria=u2 ~= 0
  Switch1 : Switch  Criteria=u2 ~= 0
  y : Outport
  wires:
  Switch1/1 -> Product/1
  Constant3/1 -> Switch1/3
  Constant2/1 -> Switch1/1
  u/1 -> Switch1/2, Switch/2
  dT/1 -> Switch/1
  Constant1/1 -> Switch/3
  Add/1 -> Product/2
  Product/1 -> Relational Operator/1, Delay/1
  Switch/1 -> Add/1
  Delay/1 -> MinMax/2
  Relational Operator/1 -> y/1
  T/1 -> MinMax/1, Relational Operator/2
  MinMax/1 -> Add/2

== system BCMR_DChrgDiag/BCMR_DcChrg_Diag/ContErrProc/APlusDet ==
  BSPR_bDCWkUp : Inport
  Enable : EnablePort  StatesWhenEnabling=reset
  Constant1 : Constant  Value=BCMR_tiDChrgHealDiagDebs_C
  Constant2 : Constant  Value=BCMR_tiDChrgDiagBase_C
  Constant4 : Constant  Value=BCMR_tiDChrgDetDiagDebs_C
  Constant7 : Constant  Value=BCMR_tiDChrgDiagBase_C
  Logical Operator1 : Logic  Operator=NOT  AllPortsSameDT=off  OutDataTypeStr=boolean
  TONV_VariableTimeDebounce1 : Subsystem  TreatAsAtomicUnit=on  RTWFcnName=TONV_VariableTimeDebounce  RTWFileName=SrvLib
  TONV_VariableTimeDebounce2 : Subsystem  TreatAsAtomicUnit=on  RTWFcnName=TONV_VariableTimeDebounce  RTWFileName=SrvLib
  BCMR_bChrgCnnttErrDet : Outport  OutputWhenDisabled=reset  InitialOutput=[0]
  BCMR_bChrgCnnttErrHeal : Outport  Port=2  OutputWhenDisabled=reset  InitialOutput=[0]
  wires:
  TONV_VariableTimeDebounce2/1(y) -> BCMR_bChrgCnnttErrHeal/1  "BCMR_bChrgCnnttErrHeal"
  TONV_VariableTimeDebounce1/1(y) -> BCMR_bChrgCnnttErrDet/1  "BCMR_bChrgCnnttErrDet"
  BSPR_bDCWkUp/1 -> TONV_VariableTimeDebounce2/1(u), Logical Operator1/1
  Logical Operator1/1 -> TONV_VariableTimeDebounce1/1(u)
  Constant7/1 -> TONV_VariableTimeDebounce1/3(dT)
  Constant4/1 -> TONV_VariableTimeDebounce1/2(T)
  Constant1/1 -> TONV_VariableTimeDebounce2/2(T)
  Constant2/1 -> TONV_VariableTimeDebounce2/3(dT)

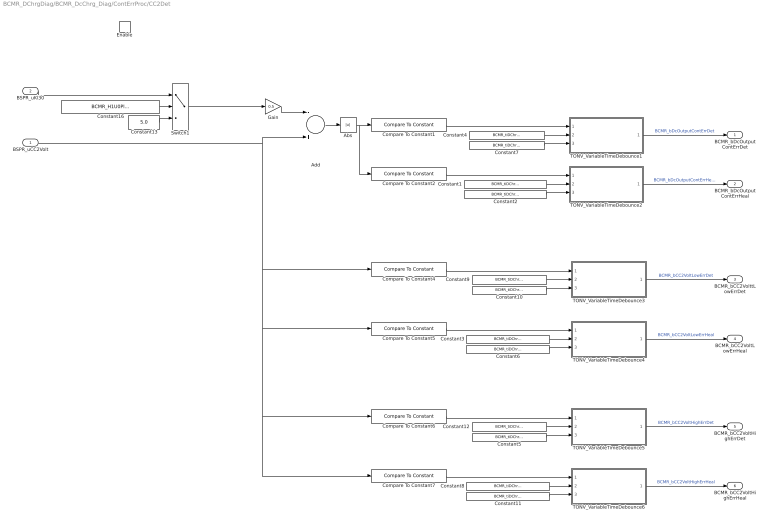
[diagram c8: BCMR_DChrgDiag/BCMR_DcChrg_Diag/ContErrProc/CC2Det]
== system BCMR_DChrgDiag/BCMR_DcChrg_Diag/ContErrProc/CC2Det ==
  BSPR_uCC2Volt : Inport
  BSPR_uKl30 : Inport  Port=2
  Enable : EnablePort  StatesWhenEnabling=reset
  Abs : Abs
  Add : Sum  Inputs=-+
  Compare To Constant1 : simulink/Logic and Bit Operations/Compare To Constant  relop=>  const=BCMR_uCC2ChkDiffDet_C  OutDataTypeStr=boolean
  Compare To Constant2 : simulink/Logic and Bit Operations/Compare To Constant  relop=<  const=BCMR_uCC2ChkDiffHeal_C  OutDataTypeStr=boolean
  Compare To Constant4 : simulink/Logic and Bit Operations/Compare To Constant  relop=<  const=BCMR_uCC2VoltLowDet_C  OutDataTypeStr=boolean
  Compare To Constant5 : simulink/Logic and Bit Operations/Compare To Constant  relop=>  const=BCMR_uCC2VoltLowHeal_C  OutDataTypeStr=boolean
  Compare To Constant6 : simulink/Logic and Bit Operations/Compare To Constant  relop=>  const=BCMR_uCC2VoltHighDet_C  OutDataTypeStr=boolean
  Compare To Constant7 : simulink/Logic and Bit Operations/Compare To Constant  relop=<  const=BCMR_uCC2VoltHighHeal_C  OutDataTypeStr=boolean
  Constant1 : Constant  Value=BCMR_tiDChrgHealDiagDebs_C
  Constant{2,5..7,10..11} (6 alike) : Constant  Value=BCMR_tiDChrgDiagBase_C
  Constant12 : Constant  Value=BCMR_tiDChrgDetDiagDebs_C
  Constant13 : Constant  Value=5.0  OutDataTypeStr=single
  Constant16 : Constant  Value=BCMR_H1U0PlatformSwDiag_C
  Constant3 : Constant  Value=BCMR_tiDChrgHealDiagDebs_C
  Constant4 : Constant  Value=BCMR_tiDChrgDetDiagDebs_C
  Constant8 : Constant  Value=BCMR_tiDChrgHealDiagDebs_C
  Constant9 : Constant  Value=BCMR_tiDChrgDetDiagDebs_C
  Gain : Gain  Gain=0.5
  Switch1 : Switch  Criteria=u2 ~= 0
  TONV_VariableTimeDebounce1 : Subsystem  TreatAsAtomicUnit=on  RTWFcnName=TONV_VariableTimeDebounce  RTWFileName=SrvLib
  TONV_VariableTimeDebounce2 : Subsystem  TreatAsAtomicUnit=on  RTWFcnName=TONV_VariableTimeDebounce  RTWFileName=SrvLib
  TONV_VariableTimeDebounce3 : Subsystem  TreatAsAtomicUnit=on  RTWFcnName=TONV_VariableTimeDebounce  RTWFileName=SrvLib
  TONV_VariableTimeDebounce4 : Subsystem  TreatAsAtomicUnit=on  RTWFcnName=TONV_VariableTimeDebounce  RTWFileName=SrvLib
  TONV_VariableTimeDebounce5 : Subsystem  TreatAsAtomicUnit=on  RTWFcnName=TONV_VariableTimeDebounce  RTWFileName=SrvLib
  TONV_VariableTimeDebounce6 : Subsystem  TreatAsAtomicUnit=on  RTWFcnName=TONV_VariableTimeDebounce  RTWFileName=SrvLib
  BCMR_bDcOutputContErrDet : Outport  OutputWhenDisabled=reset  InitialOutput=[0]
  BCMR_bDcOutputContErrHeal : Outport  Port=2  OutputWhenDisabled=reset  InitialOutput=[0]
  BCMR_bCC2VolttLowErrDet : Outport  Port=3  OutputWhenDisabled=reset  InitialOutput=[0]
  BCMR_bCC2VoltLowErrHeal : Outport  Port=4  OutputWhenDisabled=reset  InitialOutput=[0]
  BCMR_bCC2VoltHighErrDet : Outport  Port=5  OutputWhenDisabled=reset  InitialOutput=[0]
  BCMR_bCC2VoltHighErrHeal : Outport  Port=6  OutputWhenDisabled=reset  InitialOutput=[0]
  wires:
  Add/1 -> Abs/1
  Abs/1 -> Compare To Constant2/1, Compare To Constant1/1
  TONV_VariableTimeDebounce2/1(y) -> BCMR_bDcOutputContErrHeal/1  "BCMR_bDcOutputContErrHeal"
  TONV_VariableTimeDebounce1/1(y) -> BCMR_bDcOutputContErrDet/1  "BCMR_bDcOutputContErrDet"
  Compare To Constant1/1 -> TONV_VariableTimeDebounce1/1(u)
  BSPR_uKl30/1 -> Switch1/1
  Gain/1 -> Add/1
  Compare To Constant4/1 -> TONV_VariableTimeDebounce3/1(u)
  Compare To Constant5/1 -> TONV_VariableTimeDebounce4/1(u)
  Constant2/1 -> TONV_VariableTimeDebounce2/3(dT)
  Constant7/1 -> TONV_VariableTimeDebounce1/3(dT)
  Constant4/1 -> TONV_VariableTimeDebounce1/2(T)
  Constant10/1 -> TONV_VariableTimeDebounce3/3(dT)
  Constant9/1 -> TONV_VariableTimeDebounce3/2(T)
  Constant6/1 -> TONV_VariableTimeDebounce4/3(dT)
  Constant3/1 -> TONV_VariableTimeDebounce4/2(T)
  BSPR_uCC2Volt/1 -> Compare To Constant7/1, Compare To Constant6/1, Compare To Constant5/1, Compare To Constant4/1, Add/2
  Compare To Constant6/1 -> TONV_VariableTimeDebounce5/1(u)
  Compare To Constant7/1 -> TONV_VariableTimeDebounce6/1(u)
  Constant5/1 -> TONV_VariableTimeDebounce5/3(dT)
  Constant12/1 -> TONV_VariableTimeDebounce5/2(T)
  Constant11/1 -> TONV_VariableTimeDebounce6/3(dT)
  Constant8/1 -> TONV_VariableTimeDebounce6/2(T)
  TONV_VariableTimeDebounce3/1(y) -> BCMR_bCC2VolttLowErrDet/1  "BCMR_bCC2VoltLowErrDet"
  TONV_VariableTimeDebounce4/1(y) -> BCMR_bCC2VoltLowErrHeal/1  "BCMR_bCC2VoltLowErrHeal"
  TONV_VariableTimeDebounce5/1(y) -> BCMR_bCC2VoltHighErrDet/1  "BCMR_bCC2VoltHighErrDet"
  TONV_VariableTimeDebounce6/1(y) -> BCMR_bCC2VoltHighErrHeal/1  "BCMR_bCC2VoltHighErrHeal"
  Constant1/1 -> TONV_VariableTimeDebounce2/2(T)
  Compare To Constant2/1 -> TONV_VariableTimeDebounce2/1(u)
  Constant16/1 -> Switch1/2
  Constant13/1 -> Switch1/3
  Switch1/1 -> Gain/1

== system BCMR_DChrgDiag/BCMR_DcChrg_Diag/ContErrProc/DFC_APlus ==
  BCMR_bChrgCnnttErrDet : Inport
  BCMR_bChrgCnnttErrHeal : Inport  Port=2
  Bitwise Operator1 : simulink/Logic and Bit Operations/Bitwise Operator  logicop=AND  UseBitMask=on  BitMask=bin2dec('00011000')  BitMaskRealWorld=Stored Integer
  Compare To Constant6 : simulink/Logic and Bit Operations/Compare To Constant  relop===  const=24  OutDataTypeStr=boolean
  DSM_ReportCheckSelfHeal : Subsystem  TreatAsAtomicUnit=on  RTWFcnName=DSM_ReportCheck  RTWFileName=SrvLib
  Data Store Read : DataStoreRead  DataStoreName=DFC_APlusChk
  Data Store Read1 : DataStoreRead  DataStoreName=DFC_APlusChk
  Data Store Write : DataStoreWrite  DataStoreName=DFC_APlusChk
  Data Type Conversion : DataTypeConversion  OutDataTypeStr=uint8
  BCMR_stDChrgCnntErr : Outport  OutputWhenDisabled=reset  InitialOutput=[0]
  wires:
  Compare To Constant6/1 -> Data Type Conversion/1
  Bitwise Operator1/1 -> Compare To Constant6/1
  DSM_ReportCheckSelfHeal/1(Dfc_id) -> Data Store Write/1
  Data Store Read/1 -> DSM_ReportCheckSelfHeal/1(Dfc_id_nv)
  Data Store Read1/1 -> Bitwise Operator1/1
  Data Type Conversion/1 -> BCMR_stDChrgCnntErr/1  "BCMR_stDChrgCnntErr"
  BCMR_bChrgCnnttErrDet/1 -> DSM_ReportCheckSelfHeal/2(Err)
  BCMR_bChrgCnnttErrHeal/1 -> DSM_ReportCheckSelfHeal/3(Heal)
